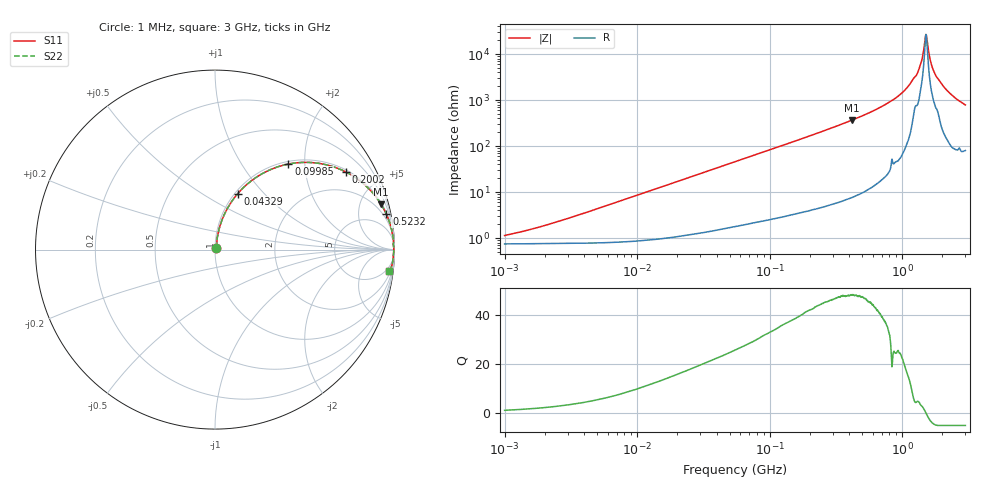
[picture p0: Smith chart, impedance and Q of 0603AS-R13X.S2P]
!s-Parameter Generated by FASTRON Sdn. Bhd.
!FASTRON P/N : 0603AS-R13X
!Keysight Technologies: E4991B_MY54100416_A.01.15
!Date created: Tue Oct 17 14:22:01 2023
!Version  : Rev01 Tue Oct 17 14:22:01 2023
!Data & Calibration Information:
!Freq	S11	S21	S12	S22
!PortZ  Port1:50+j0  Port2:50+j0
!When reading reference impedance value at option line is always used.
! Remarks : This data is being provided solely for informational purposes.
# Hz S dB R 50
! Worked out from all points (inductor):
!   1601 points, 1 MHz to 3 GHz, reference 50 ohm
!   read as one part in series: L = 137 nH near 2.68 MHz
!   highest Q = 48 at 415.6 MHz (marker M1), where L = 140 nH
!   self-resonance near 1.511 GHz
!   S11 on the Smith chart (normalised r, x): 1 MHz: 1.02, +0.02; 43.29 MHz: 1.03, +0.72; 99.85 MHz: 1.05, +1.65; 200.2 MHz: 1.08, +3.33; 523.2 MHz: 1.21, +9.64; 3 GHz: 3, -16
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1000000  -38.89 48.5  -0.07 -0.5  -0.07 -0.5  -38.89 48.5
3804036  -29.56 74.7  -0.07 -1.9  -0.07 -1.9  -29.56 74.7
1.447069e7  -18.33 78.6  -0.15 -6.9  -0.15 -6.9  -18.33 78.6
4.329325e7  -9.47 67.9  -0.65 -19.6  -0.65 -19.6  -9.47 67.9
5.477226e7  -7.76 63.6  -0.95 -24.2  -0.95 -24.2  -7.76 63.6
9.984923e7  -4.04 49.4  -2.39 -38.9  -2.39 -38.9  -4.04 49.4
2.001795e8  -1.43 30.6  -5.86 -58.0  -5.86 -58.0  -1.43 30.6
2.083556e8  -1.33 29.6  -6.12 -59.0  -6.12 -59.0  -1.33 29.6
4.156301e8  -0.36 15.2  -11.61 -73.6  -11.61 -73.6  -0.36 15.2
5.232078e8  -0.22 11.7  -13.88 -77.1  -13.88 -77.1  -0.22 11.7
7.925923e8  -0.08 6.4  -19.09 -81.9  -19.09 -81.9  -0.08 6.4
1.033307e9  -0.04 3.6  -24.05 -83.5  -24.05 -83.5  -0.04 3.6
1.274982e9  -0.06 1.6  -30.71 -75.5  -30.71 -75.5  -0.06 1.6
1.374365e9  -0.04 0.9  -35.44 -72.9  -35.44 -72.9  -0.04 0.9
1.474099e9  -0.03 0.3  -44.30 -51.0  -44.30 -51.0  -0.03 0.3
1.511446e9  -0.03 0.0  -48.56 -5.0  -48.56 -5.0  -0.03 0.0
1.557514e9  -0.03 -0.3  -44.14 52.0  -44.14 52.0  -0.03 -0.3
1.629261e9  -0.04 -0.7  -37.45 71.2  -37.45 71.2  -0.04 -0.7
1.67892e9  -0.04 -1.0  -34.70 74.4  -34.70 74.4  -0.04 -1.0
1.827992e9  -0.06 -1.8  -29.98 76.7  -29.98 76.7  -0.06 -1.8
2.266846e9  -0.07 -3.9  -23.29 81.6  -23.29 81.6  -0.07 -3.9
3e9  -0.18 -7.1  -18.08 77.0  -18.08 77.0  -0.18 -7.1
